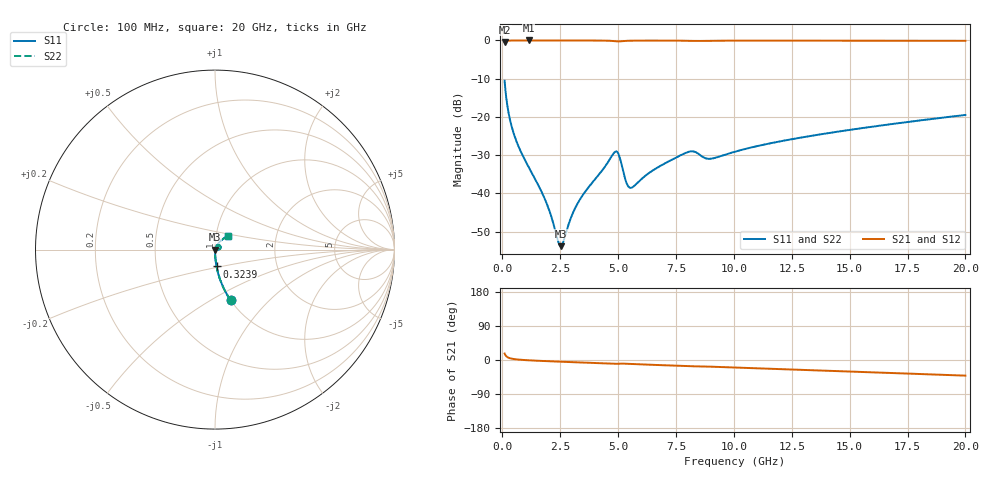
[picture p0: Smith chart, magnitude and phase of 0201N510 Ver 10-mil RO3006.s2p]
# GHz S MA R 50
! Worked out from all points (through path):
!   1601 points, 100 MHz to 20 GHz, reference 50 ohm
!   highest |S21| = -0.01 dB at 1.132 GHz (marker M1); lowest = -0.4 dB at 100 MHz (marker M2)
!   group delay of S21, straight-line fit = 5.95 ps
!   lowest |S11| = -53.8 dB at 2.525 GHz (marker M3), VSWR 1.00, Z = 50.2 - j0.0261 ohm
!   |S11| at or under -10 dB: start of sweep to end of sweep
!   |S22| runs from -53.8 to -10.6 dB; largest |S21 - S12| = 0
!   S11 on the Smith chart (normalised r, x): 100 MHz: 1.00, -0.62; 323.9 MHz: 1.00, -0.19; 20 GHz: 1.15, +0.17
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0.1  0.2967 -72.8  0.9543 17.1  0.9543 17.1  0.2967 -72.8
0.323875  0.09415 -84.7  0.9948 4.8  0.9948 4.8  0.09415 -84.7
0.622375  0.04706 -87.3  0.9979 1.6  0.9979 1.6  0.04706 -87.3
1.132313  0.02224 -87.5  0.9984 -0.8  0.9984 -0.8  0.02224 -87.5
1.866125  0.008038 -80.7  0.9982 -2.9  0.9982 -2.9  0.008038 -80.7
2.102438  0.005128 -72.8  0.9981 -3.5  0.9981 -3.5  0.005128 -72.8
2.413375  0.002351 -37.0  0.998 -4.3  0.998 -4.3  0.002351 -37.0
2.525313  0.002038 -7.3  0.9979 -4.5  0.9979 -4.5  0.002038 -7.3
2.63725  0.002339 21.5  0.9978 -4.8  0.9978 -4.8  0.002339 21.5
3.047687  0.005528 59.2  0.9976 -5.8  0.9976 -5.8  0.005528 59.2
3.420812  0.008959 66.3  0.9972 -6.6  0.9972 -6.6  0.008959 66.3
4.876  0.03502 37.2  0.9759 -10.2  0.9759 -10.2  0.03502 37.2
5.02525  0.03231 14.9  0.9704 -9.8  0.9704 -9.8  0.03231 14.9
5.348625  0.01409 8.7  0.9865 -9.9  0.9865 -9.9  0.01409 8.7
5.52275  0.01182 28.6  0.9906 -10.3  0.9906 -10.3  0.01182 28.6
6.741625  0.02211 63.8  0.9947 -13.3  0.9947 -13.3  0.02211 63.8
8.097312  0.0352 53.3  0.987 -16.4  0.987 -16.4  0.0352 53.3
8.930625  0.02827 49.8  0.9885 -17.5  0.9885 -17.5  0.02827 49.8
10.05  0.03505 60.3  0.9932 -19.9  0.9932 -19.9  0.03505 60.3
13.37081  0.05668 57.6  0.9928 -27.0  0.9928 -27.0  0.05668 57.6
16.69162  0.07961 51.8  0.9907 -34.1  0.9907 -34.1  0.07961 51.8
20  0.106 45.3  0.9876 -41.2  0.9876 -41.2  0.106 45.3
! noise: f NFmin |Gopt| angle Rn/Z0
0.1  0.000505  0.9157  0.2491  0.001321
2.301  0.004164  0.7813  4.145  0.003899
4.515  0.0115  0.8398  8.094  0.01514
6.729  0.01139  0.7688  12.03  0.009928
8.943  0.01941  0.8156  15.97  0.02158
11.14  0.01524  0.7232  19.76  0.01061
13.36  0.01667  0.702  23.56  0.01052
15.57  0.01847  0.6905  27.32  0.01099
17.79  0.02035  0.6826  31.03  0.01156
20  0.02225  0.6769  34.69  0.01215
